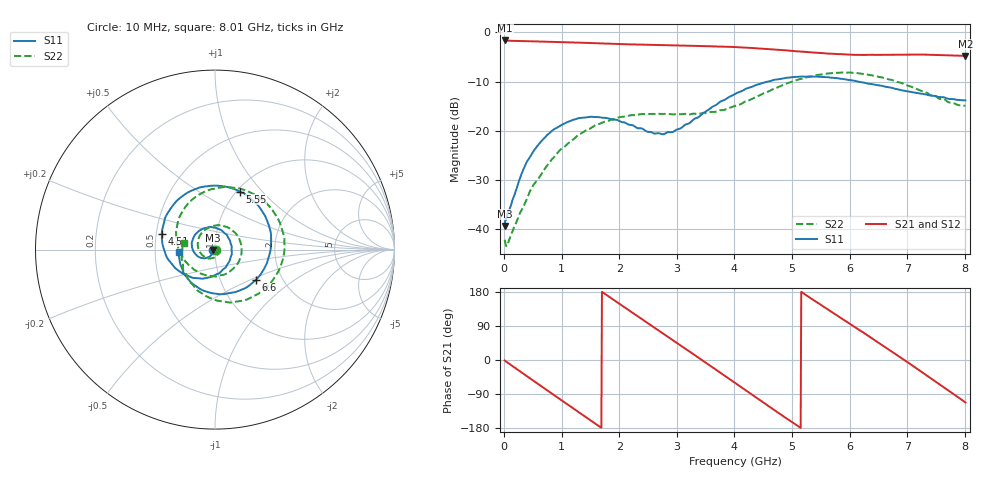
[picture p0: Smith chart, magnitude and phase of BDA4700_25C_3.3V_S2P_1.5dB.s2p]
!Agilent Technologies,E5071B,MY42404982,A.09.10
!Date: Mon Oct 20 18:03:36 2025
!Data & Calibration Information:
!Freq	S11:SOLT2(ON)	S21:SOLT2(ON)	S12:SOLT2(ON)	S22:SOLT2(ON)
# Hz S RI R 50
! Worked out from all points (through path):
!   801 points, 10 MHz to 8.01 GHz, reference 50 ohm
!   highest |S21| = -1.62 dB at 20 MHz (marker M1); lowest = -4.8 dB at 8.01 GHz (marker M2)
!   group delay of S21, straight-line fit = 287 ps
!   lowest |S11| = -39.3 dB at 10 MHz (marker M3), VSWR 1.02, Z = 49 - j0.201 ohm
!   |S11| at or under -10 dB: start of sweep to 4.58 GHz; 6.151 GHz to end of sweep
!   |S22| runs from -43.5 to -8.1 dB; largest |S21 - S12| = 0.0091
!   S11 on the Smith chart (normalised r, x): 10 MHz: 0.98, -0.00; 4.51 GHz: 0.54, +0.11; 5.55 GHz: 1.03, +0.76; 6.6 GHz: 1.47, -0.54; 8.01 GHz: 0.66, -0.02
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1e7  -0.0106 -0.00205  0.829 -0.0176  0.829 -0.0187  0.00771 -0.00106
2e7  -0.0116 -0.00369  0.8288 -0.0326  0.8285 -0.0348  0.00743 7.64e-05
3.7e8  -0.0267 -0.0362  0.6271 -0.522  0.6264 -0.5225  0.0155 -0.0105
7.2e8  -0.0732 -0.047  0.1822 -0.785  0.1822 -0.7849  -0.00118 -0.0422
1.02e9  -0.1152 -0.0172  -0.2536 -0.7557  -0.2542 -0.7556  -0.0493 -0.0453
1.35e9  -0.1273 0.0462  -0.6309 -0.4693  -0.6309 -0.4697  -0.094 0.0109
1.92e9  -0.0357 0.1249  -0.7054 0.2999  -0.7058 0.2997  -0.00742 0.1326
2.32e9  0.0513 0.093  -0.3247 0.6797  -0.3246 0.6799  0.1131 0.0926
2.68e9  0.0926 0.0193  0.1515 0.7298  0.1503 0.7292  0.1469 -0.0252
3.36e9  0.0126 -0.1356  0.7227 0.0983  0.7235 0.0984  -0.0125 -0.1477
3.67e9  -0.0859 -0.1599  0.6558 -0.3002  0.6557 -0.3021  -0.0973 -0.1221
4.01e9  -0.2068 -0.1154  0.3514 -0.6179  0.3524 -0.617  -0.1683 -0.0609
4.51e9  -0.2967 0.0891  -0.2669 -0.6298  -0.2666 -0.631  -0.2166 0.1052
4.93e9  -0.1994 0.2839  -0.6023 -0.2593  -0.6015 -0.2625  -0.1282 0.2782
5.35e9  0.0248 0.3551  -0.5906 0.2104  -0.5915 0.2072  0.1 0.3452
5.55e9  0.138 0.3236  -0.473 0.3915  -0.474 0.3909  0.2204 0.3074
6.07e9  0.3111 0.0926  0.0147 0.5923  0.0145 0.5952  0.3871 0.0305
6.6e9  0.2263 -0.1698  0.482 0.346  0.4826 0.344  0.2401 -0.2468
6.68e9  0.1942 -0.1975  0.5254 0.274  0.5268 0.2731  0.1986 -0.2676
7.24e9  -0.054 -0.2325  0.5141 -0.3023  0.5134 -0.3023  -0.0725 -0.2444
7.63e9  -0.1716 -0.137  0.186 -0.5575  0.1852 -0.5583  -0.1771 -0.1129
8.01e9  -0.2032 -0.0145  -0.2157 -0.5362  -0.2141 -0.5374  -0.1751 0.038
